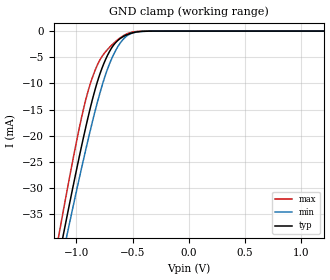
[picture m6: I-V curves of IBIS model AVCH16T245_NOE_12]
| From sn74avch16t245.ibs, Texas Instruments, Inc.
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[Model]   AVCH16T245_NOE_12
Model_type  Input
Vinl=0.385
Vinh=0.845
| variable   typ   min   max
C_comp   2.98pF   2.56pF   3.38pF
[Temperature Range]   40   100   -40
| Ambient temperature   25   85   -40
[Voltage range]   1.2   1.1   1.3
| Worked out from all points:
|   GND clamp passes 1 mA (typ) near -0.58 V on its own axis
[GND Clamp]
| AVCH16T245_NOE_12
|   Voltage   I(typ)   I(min)   I(max)
-4.6V     -463.5mA   -440.8mA   -490.1mA
-1.16V    -43.79mA   -46.85mA   -39.57mA
-1.11V    -38.33mA   -41.71mA   -33.68mA
-1.085V   -35.63mA   -39.17mA   -30.78mA
-1.06V    -32.96mA   -36.65mA   -27.92mA
-940mV    -20.66mA   -24.91mA   -15.24mA
-850mV    -12.51mA   -16.73mA   -8.451mA
-780mV    -7.568mA   -11.08mA   -5.137mA
-705mV    -3.908mA   -6.259mA   -3.112mA
-555mV    -754.1uA   -997.4uA   -574.9uA
-350mV    -10.22uA   -15.02uA   -1.919uA
1.2V      129.2pA    829.5pA    20.47pA
